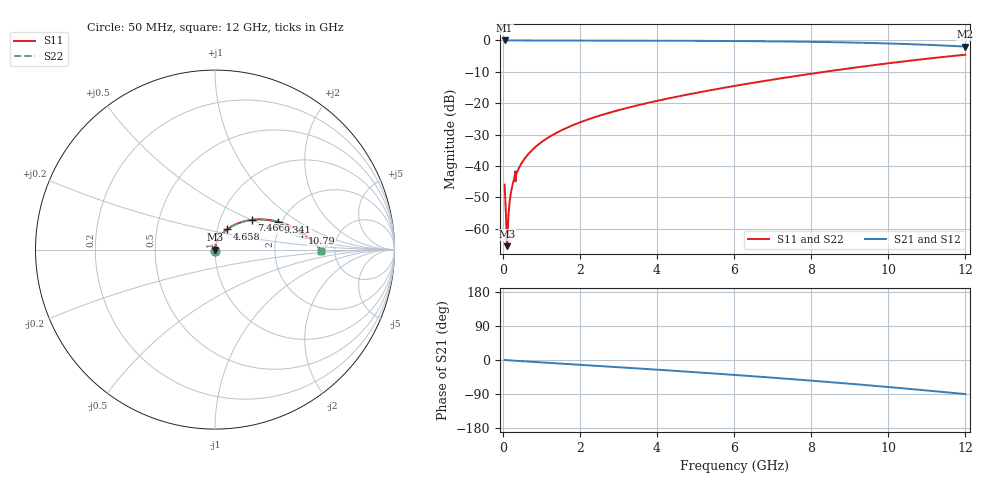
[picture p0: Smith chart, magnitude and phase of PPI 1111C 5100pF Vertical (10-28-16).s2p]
# GHz S MA R 50
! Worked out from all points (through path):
!   1601 points, 50 MHz to 12 GHz, reference 50 ohm
!   highest |S21| = 0.00 dB at 50 MHz (marker M1); lowest = -2.0 dB at 12 GHz (marker M2)
!   group delay of S21, straight-line fit = 20.5 ps
!   lowest |S11| = -65.5 dB at 109.8 MHz (marker M3), VSWR 1.00, Z = 50 - j0.02 ohm
!   |S11| at or under -10 dB: start of sweep to 8.341 GHz
!   |S22| runs from -65.5 to -4.5 dB; largest |S21 - S12| = 0
!   S11 on the Smith chart (normalised r, x): 50 MHz: 1.00, -0.01; 4.658 GHz: 1.12, +0.26; 7.466 GHz: 1.41, +0.50; 9.341 GHz: 1.92, +0.70; 10.79 GHz: 2.76, +0.68; 12 GHz: 3.92, -0.08
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0.05  0.005047 -85.8  0.9996 0.0  0.9996 0.0  0.005047 -85.8
0.079875  0.002027 -77.9  0.9996 -0.3  0.9996 -0.3  0.002027 -77.9
0.10975  0.0005299 -22.2  0.9995 -0.5  0.9995 -0.5  0.0005299 -22.2
0.1321563  0.0009834 56.7  0.9995 -0.7  0.9995 -0.7  0.0009834 56.7
0.1545625  0.001803 70.9  0.9994 -0.9  0.9994 -0.9  0.001803 70.9
0.2068437  0.003553 78.4  0.9993 -1.2  0.9993 -1.2  0.003553 78.4
0.2665938  0.00537 80.7  0.9993 -1.6  0.9993 -1.6  0.00537 80.7
0.4309062  0.009573 82.2  0.9991 -2.6  0.9991 -2.6  0.009573 82.2
0.6026875  0.01397 82.1  0.9989 -3.7  0.9989 -3.7  0.01397 82.1
0.8491562  0.02012 81.4  0.9986 -5.3  0.9986 -5.3  0.02012 81.4
1.162844  0.02794 80.0  0.9982 -7.3  0.9982 -7.3  0.02794 80.0
2.044156  0.05063 75.2  0.9968 -12.8  0.9968 -12.8  0.05063 75.2
2.918  0.07501 70.0  0.9949 -18.4  0.9949 -18.4  0.07501 70.0
4.038312  0.1104 63.0  0.9911 -25.7  0.9911 -25.7  0.1104 63.0
4.658219  0.1325 58.9  0.9881 -29.9  0.9881 -29.9  0.1325 58.9
6.025  0.1893 49.5  0.9782 -39.4  0.9782 -39.4  0.1893 49.5
7.466469  0.2634 38.9  0.9603 -50.2  0.9603 -50.2  0.2634 38.9
8.019156  0.2961 34.6  0.9504 -54.6  0.9504 -54.6  0.2961 34.6
9.341125  0.384 23.7  0.9178 -65.5  0.9178 -65.5  0.384 23.7
10.01331  0.4337 17.9  0.8951 -71.4  0.8951 -71.4  0.4337 17.9
10.79006  0.4943 10.9  0.8628 -78.5  0.8628 -78.5  0.4943 10.9
12  0.5933 -0.6  0.7976 -90.0  0.7976 -90.0  0.5933 -0.6
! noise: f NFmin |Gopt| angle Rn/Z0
0.05  0.0004128  0.8784  0.2458  0.0007345
1.372  0.004374  0.7137  6.555  0.003004
2.701  0.007264  0.6715  12.74  0.004205
4.031  0.009907  0.6499  18.76  0.005239
5.36  0.0125  0.6398  24.57  0.006267
6.682  0.01513  0.6379  30.14  0.007372
8.012  0.01794  0.6426  35.52  0.008653
9.341  0.02103  0.6532  40.7  0.01021
10.67  0.02454  0.6693  45.69  0.0122
12  0.0288  0.6914  50.55  0.01497
